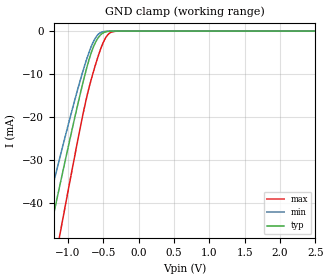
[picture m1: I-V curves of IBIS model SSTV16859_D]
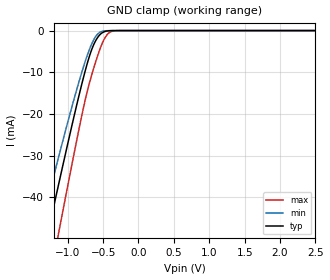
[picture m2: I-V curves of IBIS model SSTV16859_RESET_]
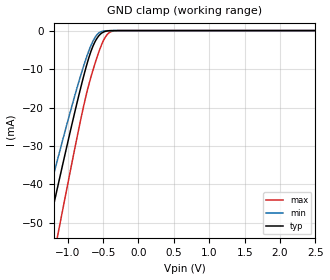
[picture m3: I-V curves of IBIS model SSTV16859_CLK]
| TEXAS INSTRUMENTS INCORPORATED
| Standard Linear and Logic Group
| IBIS Model of sn74sstv16859
| 13-Bit to 26-Bit Registered Buffer with SSTL_2 Inputs and Outputs
| This file contains package information for the following:
|  TSSOP 64-pin (DGG) package as [Component] SSTV16859_DGG
| This device can be powered at the following Vccs:
|  2.5 volt Vcc
| This file provides unique models under the [Model Selector] for each Vcc.
| For operation at a specific Vcc, select the appropriate model after each
| [Model Selector] keyword.
[IBIS Ver]   3.2
[Comment char]  |_char
[File Name]   sn74sstv16859.ibs
[File Rev]   2.1 | E_die
[Date]   February 13, 2002
[Source]   Data created from TI-SPICE simulations at TI-SLL.
[Notes]   The following is an IBIS list for the SSTV16859.
   Please contact sllibis@ti.com with questions and
   comments concerning SLL IBIS models.
   -As there is no power clamp diode in the Input model,
   we removed the Pwr Clamp table data from the Input model
   -For differential type input Vinl and Vinh should be
   set as optional, but since IBIS pursers give error, we
   set dummy values of Vinh and Vinl
[Disclaimer] Property of Texas Instruments Incorporated.  Unauthorized
   reproduction and/or distribution is strictly prohibited.
   This product is protected under copyright law.
   Created  2002, (C) Copyright  2002, Texas Instruments
   Incorporated, All Rights Reserved
   UNLESS THERE IS A SIGNED, WRITTEN AGREEMENT TO THE
   CONTRARY, TEXAS INSTRUMENTS (TI) IS PROVIDING THE IBIS
   MODELS  AND WITHOUT ANY WARRANTY, EXPRESSED OR
   IMPLIED.  TI assumes no liability for:
   1) the accuracy of the IBIS models provided to your
   company;
   2) the proper functioning of these IBIS Models in your
   design or for any resulting applications; or
   3) infringement of patents, copyrights or intellectual
   property rights resulting from your use of these IBIS
   models.
   TI provides IBIS Models as a service to our customers.
   You and your company shall not distribute, sell or give
   these models to anyone else without prior written
   permission from TI.
   TI reserves the right to make changes to our products or
   to discontinue any semiconductor product or service
   without notice, and advises our customers to obtain the
   latest version of relevant information to verify, before
   placing orders, that the information being relied on is
   current.
   Please be aware that your receipt and use of the IBIS
   information provided shall serve as acceptance of these
   terms and conditions.  If you do not accept these terms,
   you should return or destroy the IBIS models and any
   other accompanying information immediately.
| Component SSTV16859_DGG 64-pin TSSOP
[Component]   SSTV16859_DGG
[Manufacturer]   Texas Instruments, Inc.
[Package]
|   typ   min   max
R_pkg   5.500e-02   4.300e-02   7.000e-02
L_pkg   3.686e-09   2.988e-09   4.882e-09
C_pkg   6.250e-13   4.220e-13   9.610e-13
[Pin]   signal_name   model_name   R_pin   L_pin   C_pin
1   Q13A   SSTV16859_Q   4.600e-02   4.878e-09   9.030e-13
2   Q12A   SSTV16859_Q   4.600e-02   4.546e-09   9.490e-13
3   Q11A   SSTV16859_Q   5.200e-02   4.386e-09   8.450e-13
4   Q10A   SSTV16859_Q   5.800e-02   4.228e-09   7.710e-13
5   Q9A   SSTV16859_Q   6.900e-02   4.189e-09   7.760e-13
6   VDDQ   POWER   7.000e-02   3.980e-09   7.760e-13
7   GND   GND   4.900e-02   3.682e-09   6.630e-13
8   Q8A   SSTV16859_Q   5.300e-02   3.630e-09   6.040e-13
9   Q7A   SSTV16859_Q   5.400e-02   3.442e-09   5.440e-13
10   Q6A   SSTV16859_Q   5.300e-02   3.324e-09   5.110e-13
11   Q5A   SSTV16859_Q   5.600e-02   3.297e-09   4.910e-13
12   Q4A   SSTV16859_Q   5.700e-02   3.220e-09   4.640e-13
13   Q3A   SSTV16859_Q   5.700e-02   3.154e-09   4.400e-13
14   Q2A   SSTV16859_Q   5.700e-02   3.096e-09   4.300e-13
15   GND   GND   6.000e-02   3.141e-09   4.380e-13
16   Q1A   SSTV16859_Q   5.900e-02   3.057e-09   4.270e-13
17   Q13B   SSTV16859_Q   5.700e-02   2.999e-09   4.230e-13
18   VDDQ   POWER   5.900e-02   3.146e-09   4.400e-13
19   Q12B   SSTV16859_Q   5.800e-02   3.109e-09   4.330e-13
20   Q11B   SSTV16859_Q   5.700e-02   3.142e-09   4.410e-13
21   Q10B   SSTV16859_Q   5.700e-02   3.219e-09   4.690e-13
22   Q9B   SSTV16859_Q   5.500e-02   3.259e-09   4.940e-13
23   Q8B   SSTV16859_Q   5.500e-02   3.339e-09   5.190e-13
24   Q7B   SSTV16859_Q   5.400e-02   3.436e-09   5.490e-13
25   Q6B   SSTV16859_Q   5.100e-02   3.492e-09   5.970e-13
26   GND   GND   5.000e-02   3.668e-09   6.700e-13
27   VDDQ   POWER   6.700e-02   3.936e-09   7.900e-13
28   Q5B   SSTV16859_Q   6.500e-02   4.111e-09   7.920e-13
29   Q4B   SSTV16859_Q   6.000e-02   4.258e-09   7.810e-13
30   Q3B   SSTV16859_Q   5.300e-02   4.392e-09   8.520e-13
31   Q2B   SSTV16859_Q   4.700e-02   4.598e-09   9.610e-13
32   Q1B   SSTV16859_Q   4.600e-02   4.882e-09   9.100e-13
33   VDDQ   POWER   4.400e-02   4.855e-09   9.000e-13
34   GND   GND   4.500e-02   4.542e-09   9.420e-13
35   D1   SSTV16859_D   5.100e-02   4.367e-09   8.360e-13
36   D2   SSTV16859_D   5.900e-02   4.230e-09   7.640e-13
37   VCC   POWER   6.700e-02   4.155e-09   7.630e-13
38   VDDQ   POWER   6.900e-02   3.958e-09   7.660e-13
39   GND   GND   5.000e-02   3.719e-09   6.670e-13
40   D3   SSTV16859_D   4.900e-02   3.493e-09   5.910e-13
41   D4   SSTV16859_D   5.200e-02   3.414e-09   5.470e-13
42   D5   SSTV16859_D   5.400e-02   3.326e-09   5.180e-13
43   GND   GND   5.400e-02   3.249e-09   4.890e-13
44   D6   SSTV16859_D   5.600e-02   3.182e-09   4.630e-13
45   VREF   SSTV16859_VREF   5.600e-02   3.112e-09   4.390e-13
46   VCC   POWER   5.500e-02   3.036e-09   4.260e-13
47   VDDQ   POWER   5.500e-02   3.045e-09   4.320e-13
48   CLK   SSTV16859_CLK   5.800e-02   3.010e-09   4.250e-13
49   CLK_   SSTV16859_CLK   5.700e-02   2.988e-09   4.220e-13
50   GND   GND   5.900e-02   3.126e-09   4.360e-13
51   RESET_   SSTV16859_RESET_   5.800e-02   3.116e-09   4.300e-13
52   D7   SSTV16859_D   5.600e-02   3.109e-09   4.350e-13
53   D8   SSTV16859_D   5.500e-02   3.176e-09   4.550e-13
54   GND   GND   5.400e-02   3.272e-09   4.810e-13
55   D9   SSTV16859_D   5.300e-02   3.333e-09   5.050e-13
56   D10   SSTV16859_D   5.100e-02   3.378e-09   5.290e-13
57   D11   SSTV16859_D   5.200e-02   3.580e-09   5.820e-13
58   GND   GND   4.800e-02   3.650e-09   6.450e-13
59   VDDQ   POWER   6.700e-02   3.899e-09   7.670e-13
60   VCC   POWER   6.900e-02   4.190e-09   7.660e-13
61   D12   SSTV16859_D   6.000e-02   4.270e-09   7.620e-13
62   D13   SSTV16859_D   5.300e-02   4.426e-09   8.350e-13
63   GND   GND   4.800e-02   4.611e-09   9.390e-13
64   VDDQ   POWER   4.300e-02   4.845e-09   8.930e-13
| NOTE:  The [Diff Pin] section is commented out because the ibischk3 program
|   currently flags it as an Error when it shouldn't
|[Diff Pin]  inv_pin   vdiff   tdelay_typ
|35   45   310mV   NA
|36   45   310mV   NA
|40   45   310mV   NA
|41   45   310mV   NA
|42   45   310mV   NA
|44   45   310mV   NA
|52   45   310mV   NA
|53   45   310mV   NA
|55   45   310mV   NA
|56   45   310mV   NA
|57   45   310mV   NA
|61   45   310mV   NA
|62   45   310mV   NA
|48   45   180mV   NA
|49   45   180mV   NA
[Diff Pin]  inv_pin   vdiff   tdelay_typ
48   49   360mV   NA
| Models and submodels in the file (5): SSTV16859_D (Input), SSTV16859_RESET_ (Input), SSTV16859_CLK (Input), SSTV16859_VREF (Input), SSTV16859_Q (Output)
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[Model]   SSTV16859_D
Model_type  Input
Vinh = 1.4
Vinl = 1.1
| variable   typ   min   max
C_comp   1.83pF   1.54pF   2.14pF
[Temperature Range]   40   85   0
| Ambient temperature   25   70   0
[Voltage range]   2.5   2.3   2.7
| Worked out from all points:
|   GND clamp passes 1 mA (typ) near -0.55 V on its own axis
[GND Clamp]
| SSTV16859_D
|   Voltage   I(typ)   I(min)   I(max)
-2.5V     -145.1mA   -126.2mA   -169.4mA
-1.38V    -56.41mA   -47.21mA   -70.86mA
-1.345V   -53.68mA   -44.83mA   -67.76mA
-1.25V    -46.3mA    -38.42mA   -59.36mA
-1.105V   -35.15mA   -28.82mA   -46.55mA
-875mV    -18.04mA   -14.32mA   -26.56mA
-730mV    -8.287mA   -6.276mA   -15.06mA
-640mV    -3.681mA   -2.459mA   -9.455mA
-545mV    -993.8uA   -422uA     -4.487mA
-440mV    -95.5uA    -30.32uA   -934.6uA
-320mV    -2.85uA    -1.072uA   -36.37uA
2.5V      313.9pA    204.4pA    3.455nA
[Model]   SSTV16859_RESET_
Model_type  Input
Vinl = 1.7
Vinh = 0.7
| variable   typ   min   max
C_comp   1.73pF   1.39pF   2.15pF
[Temperature Range]   40   85   0
| Ambient temperature   25   70   0
[Voltage range]   2.5   2.3   2.7
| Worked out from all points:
|   GND clamp passes 1 mA (typ) near -0.55 V on its own axis
[GND Clamp]
| SSTV16859_RESET_
|   Voltage   I(typ)   I(min)   I(max)
-2.5V     -145.1mA   -126.2mA   -169.4mA
-1.42V    -59.54mA   -49.94mA   -74.39mA
-1.38V    -56.41mA   -47.21mA   -70.86mA
-1.26V    -47.07mA   -39.09mA   -60.24mA
-1.12V    -36.3mA    -29.8mA    -47.88mA
-890mV    -19.12mA   -15.22mA   -27.83mA
-735mV    -8.591mA   -6.524mA   -15.41mA
-635mV    -3.485mA   -2.293mA   -9.171mA
-540mV    -908.9uA   -375.9uA   -4.259mA
-440mV    -95.5uA    -30.32uA   -934.6uA
-325mV    -3.339uA   -1.24uA    -42.7uA
2.5V      313.9pA    204.4pA    3.455nA
[Model]   SSTV16859_CLK
Model_type  Input
Vinh = 1.53
Vinl = 0.97
| variable   typ   min   max
C_comp   2.17pF   1.83pF   2.48pF
[Temperature Range]   40   85   0
| Ambient temperature   25   70   0
[Voltage range]   2.5   2.3   2.7
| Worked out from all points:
|   GND clamp passes 1 mA (typ) near -0.54 V on its own axis
[GND Clamp]
| SSTV16859_CLK
|   Voltage   I(typ)   I(min)   I(max)
-2.5V     -148.6mA   -129.3mA   -174.2mA
-1.43V    -64.63mA   -54.2mA    -80.68mA
-1.37V    -59.6mA    -49.81mA   -74.98mA
-1.28V    -52.09mA   -43.29mA   -66.44mA
-1.14V    -40.51mA   -33.31mA   -53.17mA
-1.115V   -38.46mA   -31.56mA   -50.8mA
-745mV    -9.842mA   -7.539mA   -17.26mA
-645mV    -4.145mA   -2.825mA   -10.43mA
-545mV    -1.057mA   -453uA     -4.795mA
-445mV    -115.5uA   -36.96uA   -1.101mA
-330mV    -4.146uA   -1.526uA   -53.12uA
2.5V      348.1pA    234pA      3.679nA
